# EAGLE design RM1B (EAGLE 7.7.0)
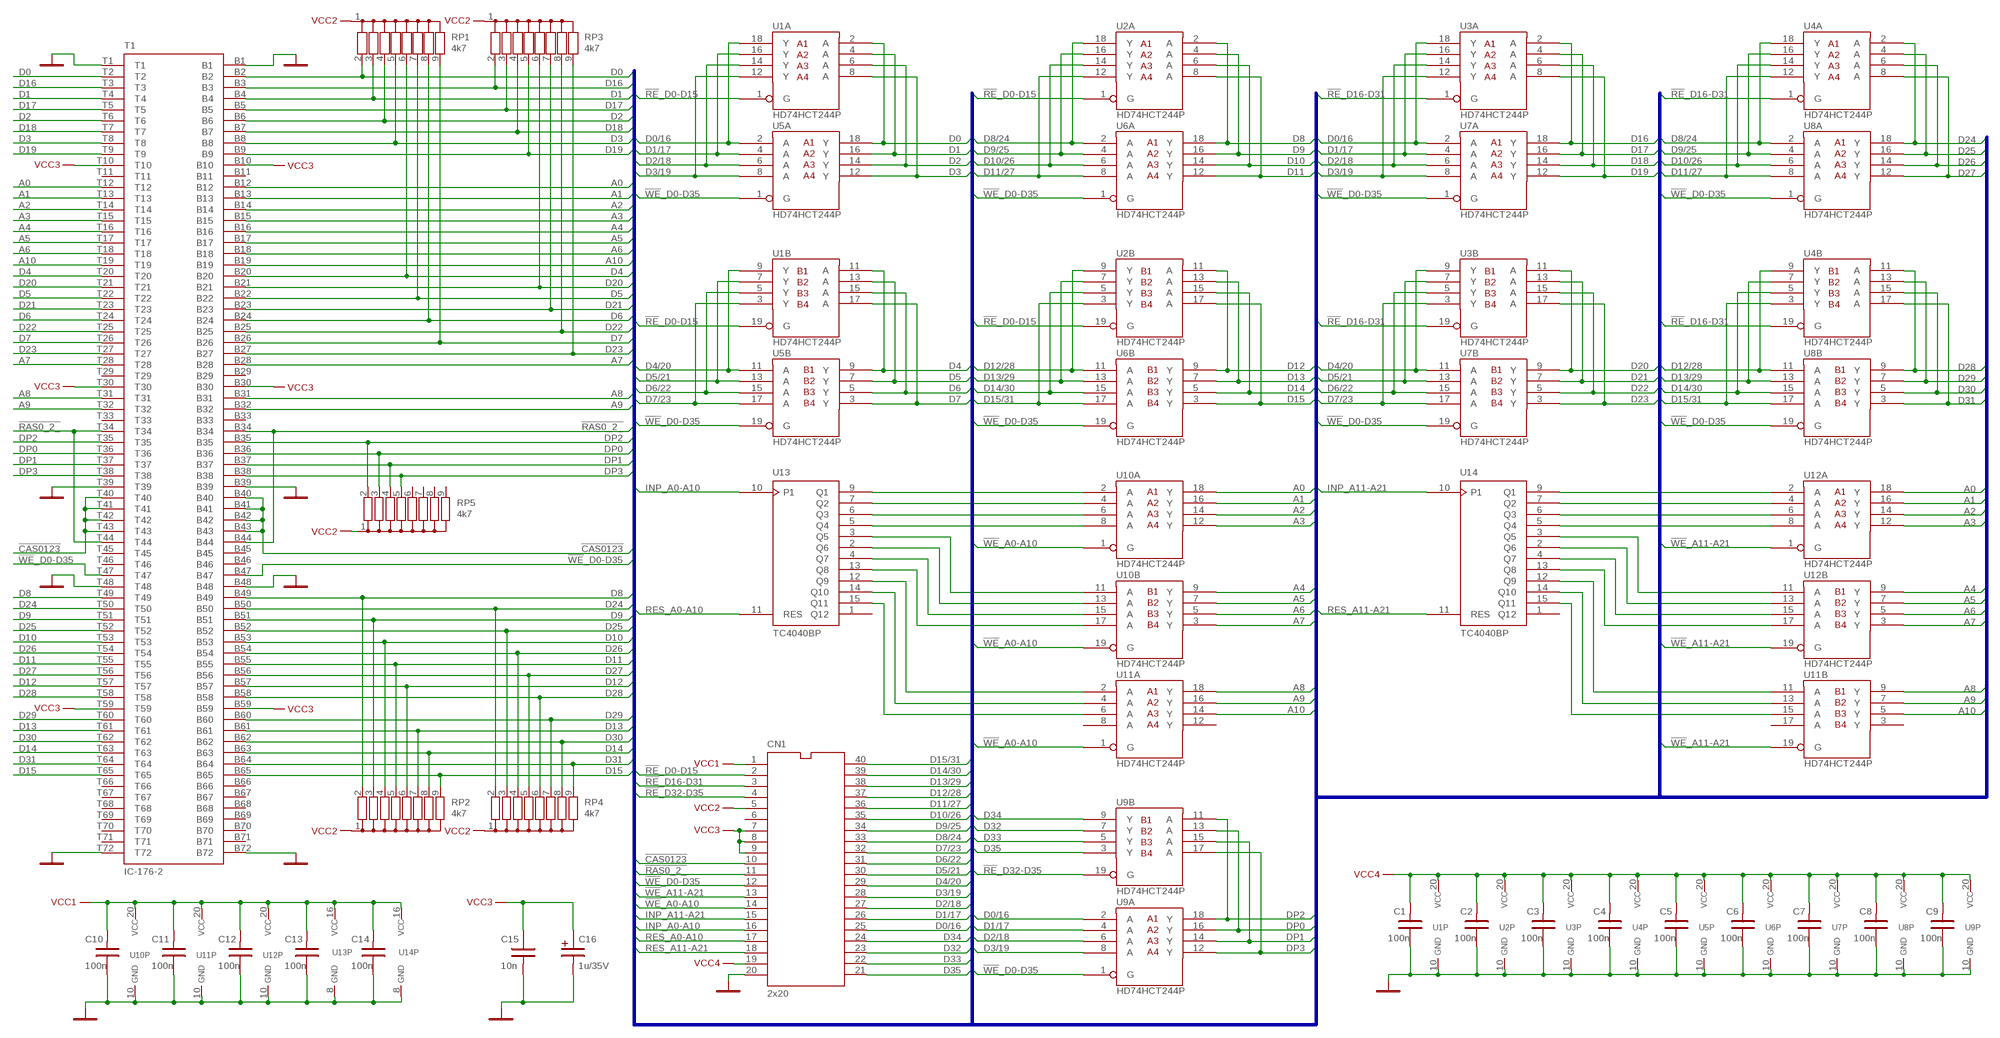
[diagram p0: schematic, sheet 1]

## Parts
C1  100n  KER-C  [KER-C]
C2  100n  KER-C  [KER-C]
C3  100n  KER-C  [KER-C]
C4  100n  KER-C  [KER-C]
C5  100n  KER-C  [KER-C]
C6  100n  KER-C  [KER-C]
C7  100n  KER-C  [KER-C]
C8  100n  KER-C  [KER-C]
C9  100n  KER-C  [KER-C]
C10  100n  KER-C  [KER-C]
C11  100n  KER-C  [KER-C]
C12  100n  KER-C  [KER-C]
C13  100n  KER-C  [KER-C]
C14  100n  KER-C  [KER-C]
C15  10n  KER-C  [KER-C]
C16  1u/35V  E-TANT-5  [E-TANT-5]
CN1  2x20  DIL40  [DIL40]
RP1  4k7  R-NET8A  [R-NET8A]
RP2  4k7  R-NET8A  [R-NET8A]
RP3  4k7  R-NET8A  [R-NET8A]
RP4  4k7  R-NET8A  [R-NET8A]
RP5  4k7  R-NET8A  [R-NET8A]
T1  IC-176-2  [IC-176-2]
U1  HD74HCT244P  74244  [DIL20]
U2  HD74HCT244P  74244  [DIL20]
U3  HD74HCT244P  74244  [DIL20]
U4  HD74HCT244P  74244  [DIL20]
U5  HD74HCT244P  74244  [DIL20]
U6  HD74HCT244P  74244  [DIL20]
U7  HD74HCT244P  74244  [DIL20]
U8  HD74HCT244P  74244  [DIL20]
U9  HD74HCT244P  74244  [DIL20]
U10  HD74HCT244P  74244  [DIL20]
U11  HD74HCT244P  74244  [DIL20]
U12  HD74HCT244P  74244  [DIL20]
U13  TC4040BP  4040  [DIL16]
U14  TC4040BP  4040  [DIL16]

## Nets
!CAS0123: CN1.10 T1.B40 T1.B41 T1.B42 T1.B43 T1.T40 T1.T41 T1.T42 T1.T43
!RAS0_2_: CN1.11 T1.B34 T1.B44 T1.T34 T1.T44
!RE!_D0-D15: CN1.2 U1.1(A:G) U1.19(B:G) U2.1(A:G) U2.19(B:G)
!RE!_D16-D31: CN1.3 U3.1(A:G) U3.19(B:G) U4.1(A:G) U4.19(B:G)
!RE!_D32-D35: CN1.4 U9.19(B:G)
!WE!_A0-A10: CN1.14 U10.1(A:G) U10.19(B:G) U11.1(A:G)
!WE!_A11-A21: CN1.13 U11.19(B:G) U12.1(A:G) U12.19(B:G)
!WE!_D0-D35: CN1.12 T1.B47 T1.T47 U5.1(A:G) U5.19(B:G) U6.1(A:G) U6.19(B:G) U7.1(A:G) U7.19(B:G) U8.1(A:G) U8.19(B:G) U9.1(A:G)
A0: T1.B12 T1.T12 U10.18(A1:Y) U12.18(A1:Y)
A1: T1.B13 T1.T13 U10.16(A2:Y) U12.16(A2:Y)
A2: T1.B14 T1.T14 U10.14(A3:Y) U12.14(A3:Y)
A3: T1.B15 T1.T15 U10.12(A4:Y) U12.12(A4:Y)
A4: T1.B16 T1.T16 U10.9(B1:Y) U12.9(B1:Y)
A5: T1.B17 T1.T17 U10.7(B2:Y) U12.7(B2:Y)
A6: T1.B18 T1.T18 U10.5(B3:Y) U12.5(B3:Y)
A7: T1.B28 T1.T28 U10.3(B4:Y) U12.3(B4:Y)
A8: T1.B31 T1.T31 U11.9(B1:Y) U11.18(A1:Y)
A9: T1.B32 T1.T32 U11.7(B2:Y) U11.16(A2:Y)
A10: T1.B19 T1.T19 U11.5(B3:Y) U11.14(A3:Y)
D0: RP1.2 T1.B2 T1.T2 U1.2(A1:A) U5.18(A1:Y)
D0/16: CN1.25 U1.18(A1:Y) U3.18(A1:Y) U5.2(A1:A) U7.2(A1:A) U9.2(A1:A)
D1: RP1.3 T1.B4 T1.T4 U1.4(A2:A) U5.16(A2:Y)
D1/17: CN1.26 U1.16(A2:Y) U3.16(A2:Y) U5.4(A2:A) U7.4(A2:A) U9.4(A2:A)
D2: RP1.4 T1.B6 T1.T6 U1.6(A3:A) U5.14(A3:Y)
D2/18: CN1.27 U1.14(A3:Y) U3.14(A3:Y) U5.6(A3:A) U7.6(A3:A) U9.6(A3:A)
D3: RP1.5 T1.B8 T1.T8 U1.8(A4:A) U5.12(A4:Y)
D3/19: CN1.28 U1.12(A4:Y) U3.12(A4:Y) U5.8(A4:A) U7.8(A4:A) U9.8(A4:A)
D4: RP1.6 T1.B20 T1.T20 U1.11(B1:A) U5.9(B1:Y)
D4/20: CN1.29 U1.9(B1:Y) U3.9(B1:Y) U5.11(B1:A) U7.11(B1:A)
D5: RP1.7 T1.B22 T1.T22 U1.13(B2:A) U5.7(B2:Y)
D5/21: CN1.30 U1.7(B2:Y) U3.7(B2:Y) U5.13(B2:A) U7.13(B2:A)
D6: RP1.8 T1.B24 T1.T24 U1.15(B3:A) U5.5(B3:Y)
D6/22: CN1.31 U1.5(B3:Y) U3.5(B3:Y) U5.15(B3:A) U7.15(B3:A)
D7: RP1.9 T1.B26 T1.T26 U1.17(B4:A) U5.3(B4:Y)
D7/23: CN1.32 U1.3(B4:Y) U3.3(B4:Y) U5.17(B4:A) U7.17(B4:A)
D8: RP2.2 T1.B49 T1.T49 U2.2(A1:A) U6.18(A1:Y)
D8/24: CN1.33 U2.18(A1:Y) U4.18(A1:Y) U6.2(A1:A) U8.2(A1:A)
D9: RP2.3 T1.B51 T1.T51 U2.4(A2:A) U6.16(A2:Y)
D9/25: CN1.34 U2.16(A2:Y) U4.16(A2:Y) U6.4(A2:A) U8.4(A2:A)
D10: RP2.4 T1.B53 T1.T53 U2.6(A3:A) U6.14(A3:Y)
D10/26: CN1.35 U2.14(A3:Y) U4.14(A3:Y) U6.6(A3:A) U8.6(A3:A)
D11: RP2.5 T1.B55 T1.T55 U2.8(A4:A) U6.12(A4:Y)
D11/27: CN1.36 U2.12(A4:Y) U4.12(A4:Y) U6.8(A4:A) U8.8(A4:A)
D12: RP2.6 T1.B57 T1.T57 U2.11(B1:A) U6.9(B1:Y)
D12/28: CN1.37 U2.9(B1:Y) U4.9(B1:Y) U6.11(B1:A) U8.11(B1:A)
D13: RP2.7 T1.B61 T1.T61 U2.13(B2:A) U6.7(B2:Y)
D13/29: CN1.38 U2.7(B2:Y) U4.7(B2:Y) U6.13(B2:A) U8.13(B2:A)
D14: RP2.8 T1.B63 T1.T63 U2.15(B3:A) U6.5(B3:Y)
D14/30: CN1.39 U2.5(B3:Y) U4.5(B3:Y) U6.15(B3:A) U8.15(B3:A)
D15: RP2.9 T1.B65 T1.T65 U2.17(B4:A) U6.3(B4:Y)
D15/31: CN1.40 U2.3(B4:Y) U4.3(B4:Y) U6.17(B4:A) U8.17(B4:A)
D16: RP3.2 T1.B3 T1.T3 U3.2(A1:A) U7.18(A1:Y)
D17: RP3.3 T1.B5 T1.T5 U3.4(A2:A) U7.16(A2:Y)
D18: RP3.4 T1.B7 T1.T7 U3.6(A3:A) U7.14(A3:Y)
D19: RP3.5 T1.B9 T1.T9 U3.8(A4:A) U7.12(A4:Y)
D20: RP3.6 T1.B21 T1.T21 U3.11(B1:A) U7.9(B1:Y)
D21: RP3.7 T1.B23 T1.T23 U3.13(B2:A) U7.7(B2:Y)
D22: RP3.8 T1.B25 T1.T25 U3.15(B3:A) U7.5(B3:Y)
D23: RP3.9 T1.B27 T1.T27 U3.17(B4:A) U7.3(B4:Y)
D24: RP4.2 T1.B50 T1.T50 U4.2(A1:A) U8.18(A1:Y)
D25: RP4.3 T1.B52 T1.T52 U4.4(A2:A) U8.16(A2:Y)
D26: RP4.4 T1.B54 T1.T54 U4.6(A3:A) U8.14(A3:Y)
D27: RP4.5 T1.B56 T1.T56 U4.8(A4:A) U8.12(A4:Y)
D28: RP4.6 T1.B58 T1.T58 U4.11(B1:A) U8.9(B1:Y)
D29: RP4.7 T1.B60 T1.T60 U4.13(B2:A) U8.7(B2:Y)
D30: RP4.8 T1.B62 T1.T62 U4.15(B3:A) U8.5(B3:Y)
D31: RP4.9 T1.B64 T1.T64 U4.17(B4:A) U8.3(B4:Y)
D32: CN1.23 U9.7(B2:Y)
D33: CN1.22 U9.5(B3:Y)
D34: CN1.24 U9.9(B1:Y)
D35: CN1.21 U9.3(B4:Y)
DP0: RP5.3 T1.B36 T1.T36 U9.13(B2:A) U9.16(A2:Y)
DP1: RP5.4 T1.B37 T1.T37 U9.14(A3:Y) U9.15(B3:A)
DP2: RP5.2 T1.B35 T1.T35 U9.11(B1:A) U9.18(A1:Y)
DP3: RP5.5 T1.B38 T1.T38 U9.12(A4:Y) U9.17(B4:A)
GND: C1.1 C2.1 C3.1 C4.1 C5.1 C6.1 C7.1 C8.1 C9.1 C10.1 C11.1 C12.1 C13.1 C14.1 C15.2 C16.K CN1.20 T1.B1 T1.B39 T1.B48 T1.B72 T1.T1 T1.T39 T1.T48 T1.T72 U1.10(P:GND) U2.10(P:GND) U3.10(P:GND) U4.10(P:GND) U5.10(P:GND) U6.10(P:GND) U7.10(P:GND) U8.10(P:GND) U9.10(P:GND) U10.10(P:GND) U11.10(P:GND) U12.10(P:GND) U13.8(GND) U14.8(GND)
INP_A0-A10: CN1.16 U13.10(P1)
INP_A11-A21: CN1.15 U14.10(P1)
N$1: U10.2(A1:A) U13.9(Q1)
N$2: U10.4(A2:A) U13.7(Q2)
N$3: U10.6(A3:A) U13.6(Q3)
N$4: U10.8(A4:A) U13.5(Q4)
N$5: U10.11(B1:A) U13.3(Q5)
N$6: U10.13(B2:A) U13.2(Q6)
N$7: U10.15(B3:A) U13.4(Q7)
N$8: U10.17(B4:A) U13.13(Q8)
N$9: U11.2(A1:A) U13.12(Q9)
N$10: U11.4(A2:A) U13.14(Q10)
N$11: U11.6(A3:A) U13.15(Q11)
N$12: U12.2(A1:A) U14.9(Q1)
N$13: U12.4(A2:A) U14.7(Q2)
N$14: U12.6(A3:A) U14.6(Q3)
N$15: U12.8(A4:A) U14.5(Q4)
N$16: U12.11(B1:A) U14.3(Q5)
N$17: U12.13(B2:A) U14.2(Q6)
N$18: U12.15(B3:A) U14.4(Q7)
N$19: U12.17(B4:A) U14.13(Q8)
N$20: U11.11(B1:A) U14.12(Q9)
N$21: U11.13(B2:A) U14.14(Q10)
N$22: U11.15(B3:A) U14.15(Q11)
RES_A0-A10: CN1.17 U13.11(RES)
RES_A11-A21: CN1.18 U14.11(RES)
VCC1: C10.2 C11.2 C12.2 C13.2 C14.2 CN1.1 U10.20(P:VCC) U11.20(P:VCC) U12.20(P:VCC) U13.16(VCC) U14.16(VCC)
VCC2: CN1.5 RP1.1 RP2.1 RP3.1 RP4.1 RP5.1
VCC3: C15.1 C16.A CN1.7 CN1.8 CN1.9 T1.B10 T1.B30 T1.B59 T1.T10 T1.T30 T1.T59
VCC4: C1.2 C2.2 C3.2 C4.2 C5.2 C6.2 C7.2 C8.2 C9.2 CN1.19 U1.20(P:VCC) U2.20(P:VCC) U3.20(P:VCC) U4.20(P:VCC) U5.20(P:VCC) U6.20(P:VCC) U7.20(P:VCC) U8.20(P:VCC) U9.20(P:VCC)
Unconnected: CN1.6 RP5.6 RP5.7 RP5.8 RP5.9 T1.B11 T1.B29 T1.B33 T1.B45 T1.B46 T1.B66 T1.B67 T1.B68 T1.B69 T1.B70 T1.B71 T1.T11 T1.T29 T1.T33 T1.T45 T1.T46 T1.T66 T1.T67 T1.T68 T1.T69 T1.T70 T1.T71 U11.3(B4:Y) U11.8(A4:A) U11.12(A4:Y) U11.17(B4:A) U13.1(Q12) U14.1(Q12)

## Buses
A[0..10],D[0..35],DP[0..3],!RE!_D0-D15,!RE!_D16-D31,!RE!_D32-D35,!CAS0123,!RAS0_2_,!WE!_D0-D35,!WE!_A11-A21,!WE!_A0-A10,INP_A11-A21,INP_A0-A10,RES_A0-A10,RES_A11-A21,D15/31,D14/30,D13/29,D12/28,D11/27,D10/26,D9/25,D8/24,D7/23,D6/22,D5/21,D4/20,D3/19,D2/18,D1/17,D0/16

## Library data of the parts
C1-C15 = PASIV:KER-C
C16 = PASIV:E-TANT-5
CN1 = SVORKY:DIL40
RP1-RP5 = PASIV:R-NET8A
T1 = CONNEC:IC-176-2
U1-U12 = 74499:74244
U13 U14 = 40XX:4040

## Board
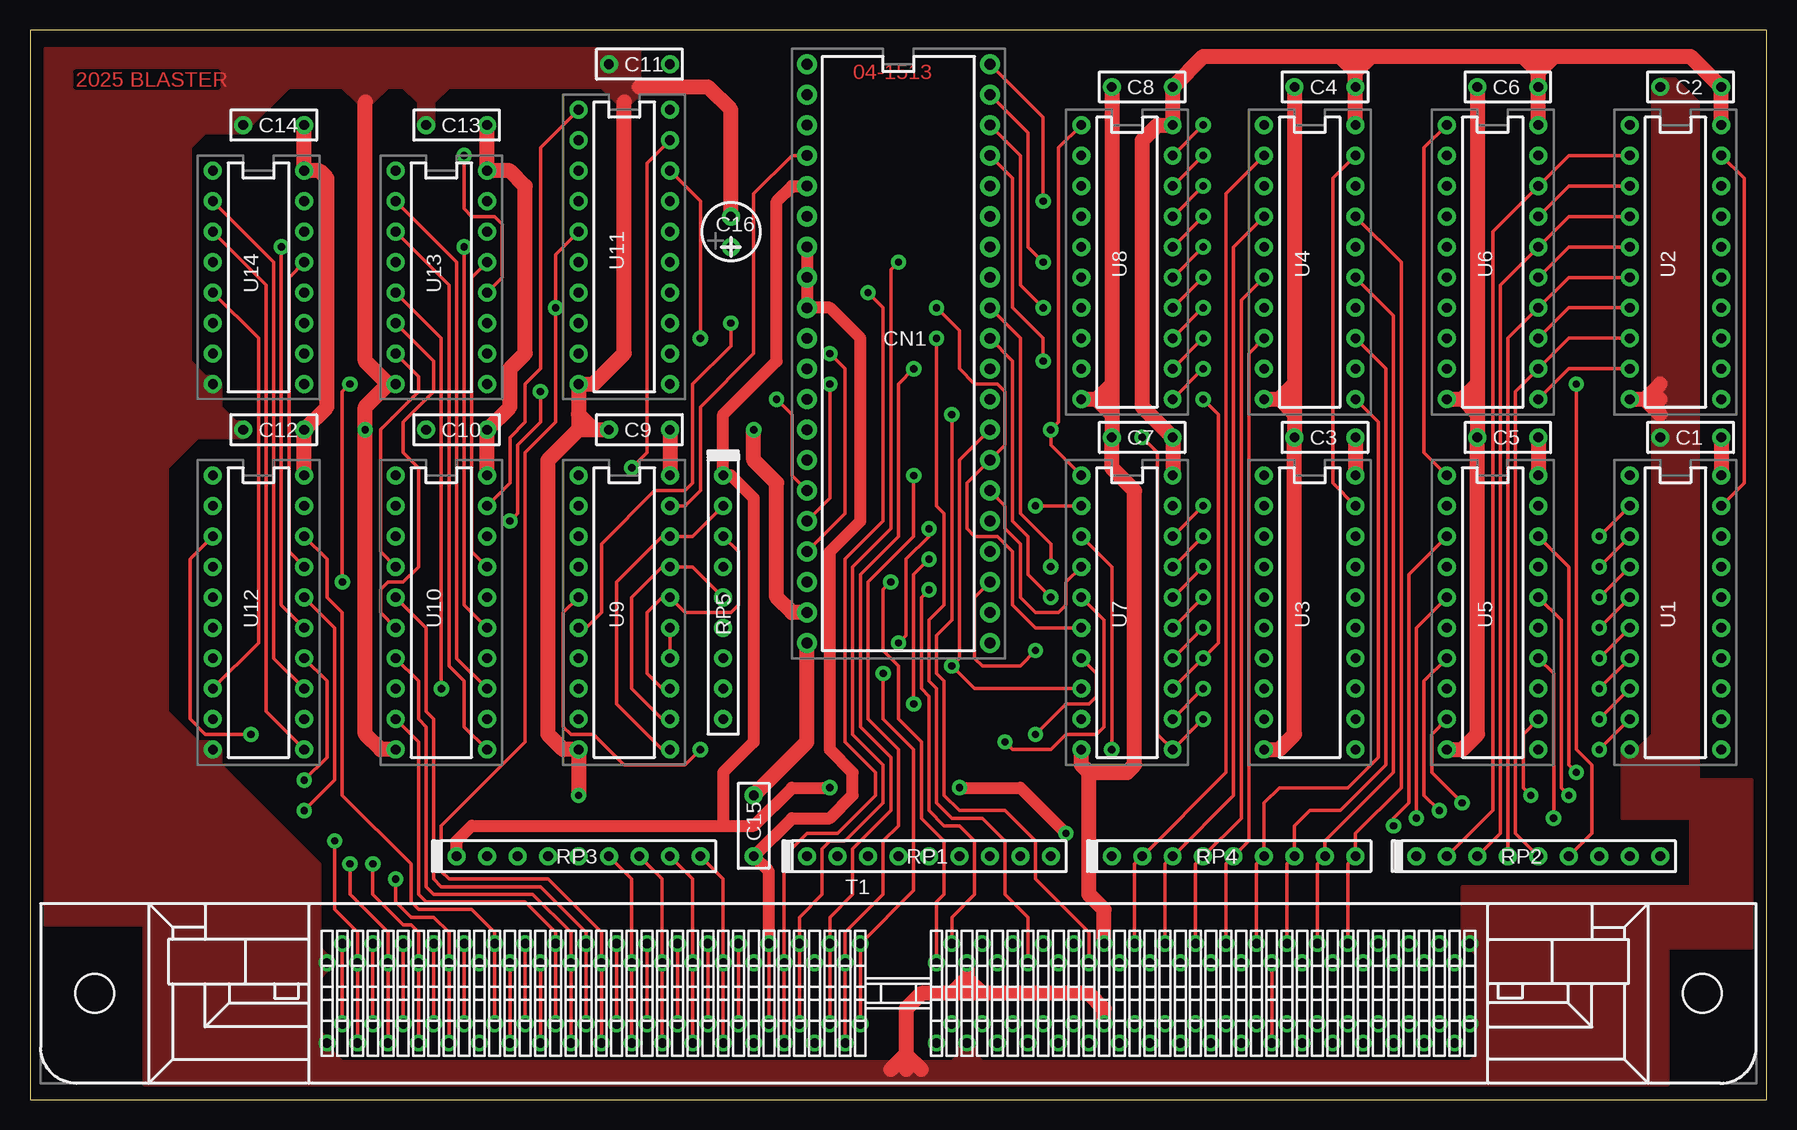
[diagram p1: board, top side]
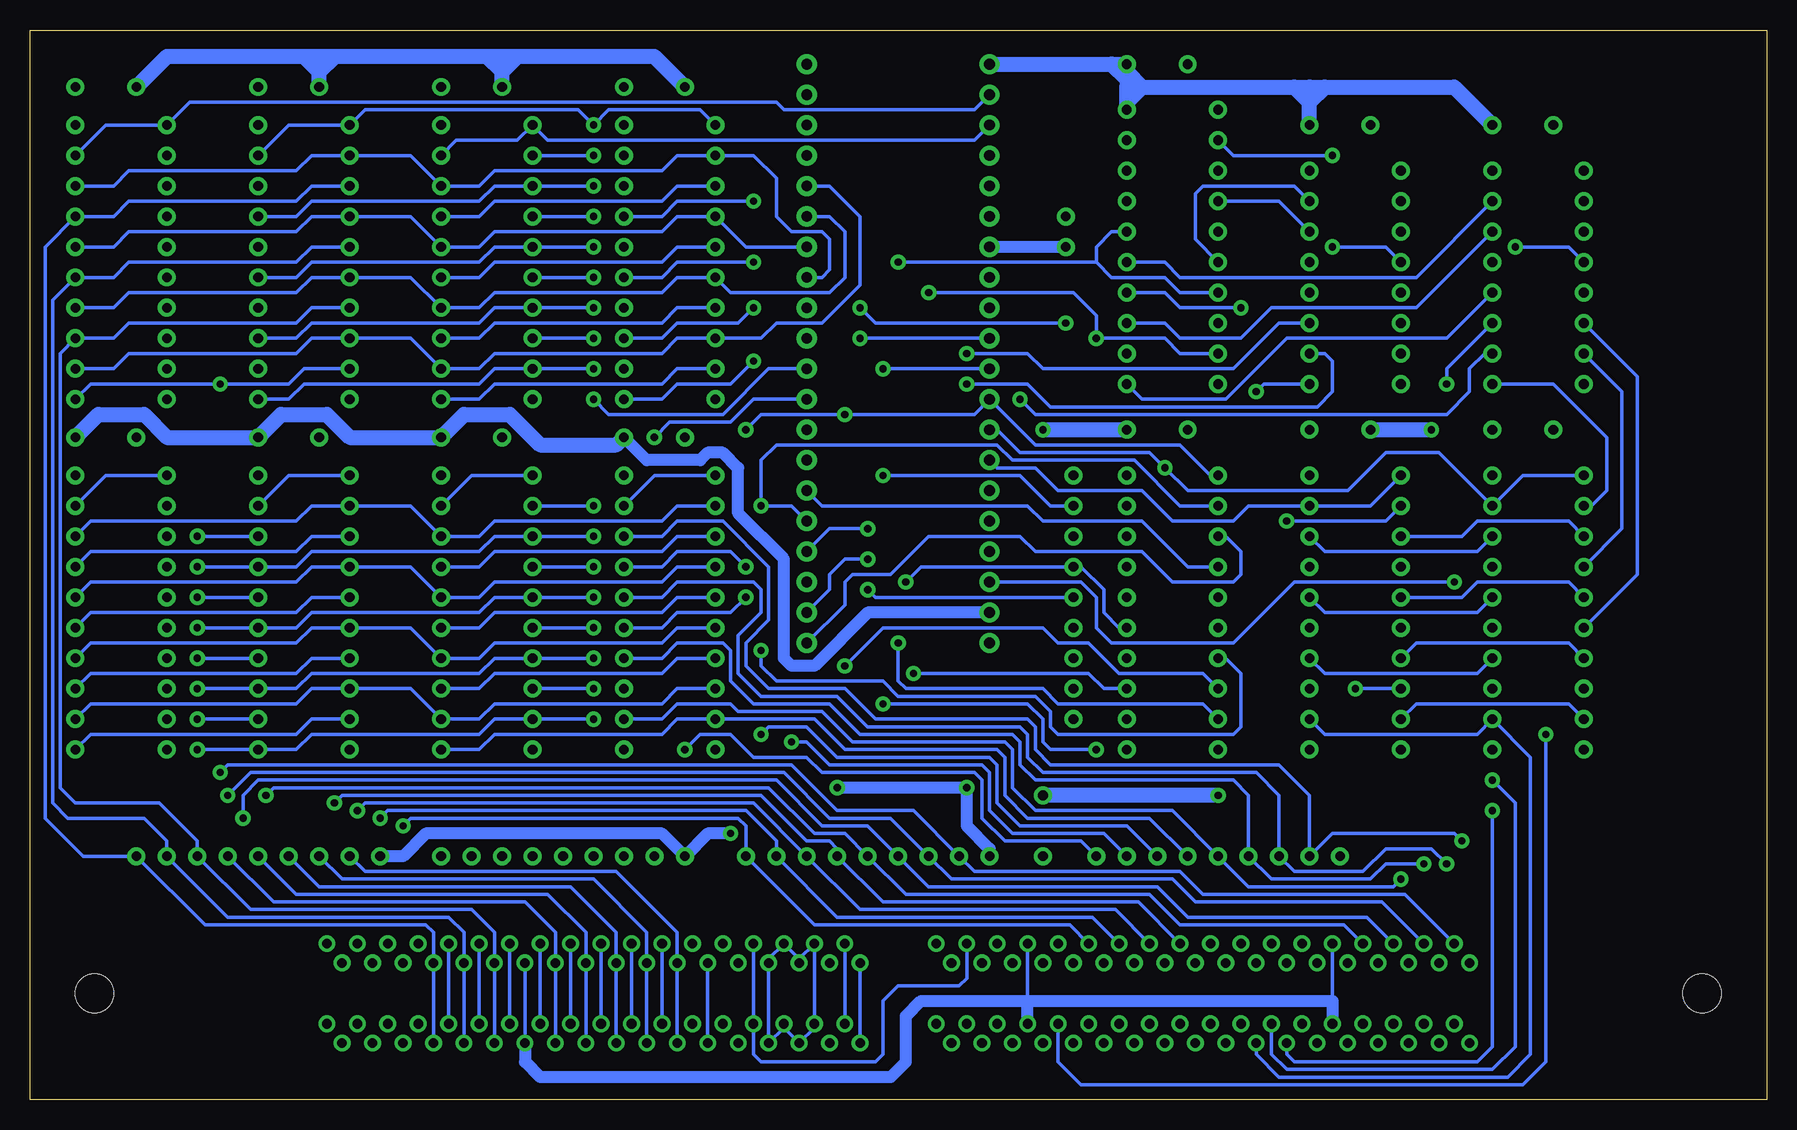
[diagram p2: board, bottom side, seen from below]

Size 144.76 x 89.2 mm. Coordinates in mm from the lower left corner, seen from the top.
Outline: 0,0 144.76,0 144.76,89.2 0,89.2 0,0
Copper layers (1*16): Top 0.035mm / dielectric 1.5mm / Bottom 0.035mm
Design rules "default *": minimum track width 10mil, minimum drill 20mil, track to track 8mil, track to pad 8mil, pad to pad 8mil, via to via 8mil, smd to smd 8mil, copper to edge 40mil, drill to drill 8mil, minimum pad ring 10mil, minimum via ring 8mil, stop-mask expansion 4mil, vias tented up to drill 0mil, thermal gap 10mil

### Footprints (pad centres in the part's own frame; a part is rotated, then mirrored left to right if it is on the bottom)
KER-C = drill 0.813 pad 1.499: 1 0,0; 2 5.08,0
E-TANT-5 = drill 0.813 pad 1.499: A -1.27,0; K 1.27,0
DIL40 = drill 0.9 pad 1.676: 1 0,0; 2 2.54,0; 3 5.08,0; 4 7.62,0; 5 10.16,0; 6 12.7,0; 7 15.24,0; 8 17.78,0; 9 20.32,0; 10 22.86,0; 11 25.4,0; 12 27.94,0; 13 30.48,0; 14 33.02,0; 15 35.56,0; 16 38.1,0; 17 40.64,0; 18 43.18,0; 19 45.72,0; 20 48.26,0; 21 48.26,15.24; 22 45.72,15.24; 23 43.18,15.24; 24 40.64,15.24; 25 38.1,15.24; 26 35.56,15.24; 27 33.02,15.24; 28 30.48,15.24; 29 27.94,15.24; 30 25.4,15.24; 31 22.86,15.24; 32 20.32,15.24; 33 17.78,15.24; 34 15.24,15.24; 35 12.7,15.24; 36 10.16,15.24; 37 7.62,15.24; 38 5.08,15.24; 39 2.54,15.24; 40 0,15.24
R-NET8A = drill 0.813 pad 1.499: 1 0,0; 2 2.54,0; 3 5.08,0; 4 7.62,0; 5 10.16,0; 6 12.7,0; 7 15.24,0; 8 17.78,0; 9 20.32,0
IC-176-2 = drill 0.8 pad 1.4: B1 -47.625,2.54; B2 -46.355,4.14; B3 -45.085,2.54; B4 -43.815,4.14; B5 -42.545,2.54; B6 -41.275,4.14; B7 -40.005,2.54; B8 -38.735,4.14; B9 -37.465,2.54; B10 -36.195,4.14; B11 -34.925,2.54; B12 -33.655,4.14; B13 -32.385,2.54; B14 -31.115,4.14; B15 -29.845,2.54; B16 -28.575,4.14; B17 -27.305,2.54; B18 -26.035,4.14; B19 -24.765,2.54; B20 -23.495,4.14; B21 -22.225,2.54; B22 -20.955,4.14; B23 -19.685,2.54; B24 -18.415,4.14; B25 -17.145,2.54; B26 -15.875,4.14; B27 -14.605,2.54; B28 -13.335,4.14; B29 -12.065,2.54; B30 -10.795,4.14; B31 -9.525,2.54; B32 -8.255,4.14; B33 -6.985,2.54; B34 -5.715,4.14; B35 -4.445,2.54; B36 -3.175,4.14; B37 3.175,2.54; B38 4.445,4.14; B39 5.715,2.54; B40 6.985,4.14; B41 8.255,2.54; B42 9.525,4.14; B43 10.795,2.54; B44 12.065,4.14; B45 13.335,2.54; B46 14.605,4.14; B47 15.875,2.54; B48 17.145,4.14; B49 18.415,2.54; B50 19.685,4.14; B51 20.955,2.54; B52 22.225,4.14; B53 23.495,2.54; B54 24.765,4.14; B55 26.035,2.54; B56 27.305,4.14; B57 28.575,2.54; B58 29.845,4.14; B59 31.115,2.54; B60 32.385,4.14; B61 33.655,2.54; B62 34.925,4.14; B63 36.195,2.54; B64 37.465,4.14; B65 38.735,2.54; B66 40.005,4.14; B67 41.275,2.54; B68 42.545,4.14; B69 43.815,2.54; B70 45.085,4.14; B71 46.355,2.54; B72 47.625,4.14; T1 -47.625,-4.14; T2 -46.355,-2.54; T3 -45.085,-4.14; T4 -43.815,-2.54; T5 -42.545,-4.14; T6 -41.275,-2.54; T7 -40.005,-4.14; T8 -38.735,-2.54; T9 -37.465,-4.14; T10 -36.195,-2.54; T11 -34.925,-4.14; T12 -33.655,-2.54; T13 -32.385,-4.14; T14 -31.115,-2.54; T15 -29.845,-4.14; T16 -28.575,-2.54; T17 -27.305,-4.14; T18 -26.035,-2.54; T19 -24.765,-4.14; T20 -23.495,-2.54; T21 -22.225,-4.14; T22 -20.955,-2.54; T23 -19.685,-4.14; T24 -18.415,-2.54; T25 -17.145,-4.14; T26 -15.875,-2.54; T27 -14.605,-4.14; T28 -13.335,-2.54; T29 -12.065,-4.14; T30 -10.795,-2.54; T31 -9.525,-4.14; T32 -8.255,-2.54; T33 -6.985,-4.14; T34 -5.715,-2.54; T35 -4.445,-4.14; T36 -3.175,-2.54; T37 3.175,-4.14; T38 4.445,-2.54; T39 5.715,-4.14; T40 6.985,-2.54; T41 8.255,-4.14; T42 9.525,-2.54; T43 10.795,-4.14; T44 12.065,-2.54; T45 13.335,-4.14; T46 14.605,-2.54; T47 15.875,-4.14; T48 17.145,-2.54; T49 18.415,-4.14; T50 19.685,-2.54; T51 20.955,-4.14; T52 22.225,-2.54; T53 23.495,-4.14; T54 24.765,-2.54; T55 26.035,-4.14; T56 27.305,-2.54; T57 28.575,-4.14; T58 29.845,-2.54; T59 31.115,-4.14; T60 32.385,-2.54; T61 33.655,-4.14; T62 34.925,-2.54; T63 36.195,-4.14; T64 37.465,-2.54; T65 38.735,-4.14; T66 40.005,-2.54; T67 41.275,-4.14; T68 42.545,-2.54; T69 43.815,-4.14; T70 45.085,-2.54; T71 46.355,-4.14; T72 47.625,-2.54 | hole 3.2: -67,0; 67,0
DIL20 = drill 0.813 pad 1.499: 1 0,0; 2 2.54,0; 3 5.08,0; 4 7.62,0; 5 10.16,0; 6 12.7,0; 7 15.24,0; 8 17.78,0; 9 20.32,0; 10 22.86,0; 11 22.86,7.62; 12 20.32,7.62; 13 17.78,7.62; 14 15.24,7.62; 15 12.7,7.62; 16 10.16,7.62; 17 7.62,7.62; 18 5.08,7.62; 19 2.54,7.62; 20 0,7.62
DIL16 = drill 0.813 pad 1.499: 1 0,0; 2 2.54,0; 3 5.08,0; 4 7.62,0; 5 10.16,0; 6 12.7,0; 7 15.24,0; 8 17.78,0; 9 17.78,7.62; 10 15.24,7.62; 11 12.7,7.62; 12 10.16,7.62; 13 7.62,7.62; 14 5.08,7.62; 15 2.54,7.62; 16 0,7.62

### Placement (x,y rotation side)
C1  135.89,55.24 0 top
C2  135.89,84.45 0 top
C3  105.41,55.24 0 top
C4  105.41,84.45 0 top
C5  120.65,55.24 0 top
C6  120.65,84.45 0 top
C7  90.17,55.24 0 top
C8  90.17,84.45 0 top
C9  48.26,55.88 0 top
C10  33.02,55.88 0 top
C11  48.26,86.36 0 top
C12  17.78,55.88 0 top
C13  33.02,81.28 0 top
C14  17.78,81.28 0 top
C15  60.33,20.32 90 top
C16  58.42,72.39 90 top
CN1  64.77,86.36 270 top
RP1  64.77,20.32 0 top
RP2  115.57,20.32 0 top
RP3  35.56,20.32 0 top
RP4  90.17,20.32 0 top
RP5  57.78,52.07 270 top
T1  72.39,8.89 0 top
U1  133.35,52.07 270 top
U2  133.35,81.28 270 top
U3  102.87,52.07 270 top
U4  102.87,81.28 270 top
U5  118.11,52.07 270 top
U6  118.11,81.28 270 top
U7  87.63,52.07 270 top
U8  87.63,81.28 270 top
U9  45.72,52.07 270 top
U10  30.48,52.07 270 top
U11  45.72,82.55 270 top
U12  15.24,52.07 270 top
U13  30.48,77.47 270 top
U14  15.24,77.47 270 top

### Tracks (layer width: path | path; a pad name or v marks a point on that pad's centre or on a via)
!CAS0123  (via drill 0.6 pad 1.27)
  Top 0.305: T1.B43 83.19,15.24 81.28,17.14 81.28,21.59 79.38,23.5 76.83,23.5 75.56,24.77 75.56,34.29 74.93,34.92 74.93,40.01 76.2,41.27 76.2,48.9 75.56,49.53 v75.56,63.5
  Bottom 0.305: T1.T42 81.92,6.02 | 81.92,6.02 T1.T43 | 81.92,6.02 T1.T41 79.38,6.02 T1.T40 T1.B40 80.64,11.76 | 80.64,11.76 T1.B42 83.19,11.76 T1.B43 83.19,4.76 | T1.B41 80.64,11.76 | v75.56,63.5 CN1.10
!RAS0_2_  (via drill 0.6 pad 1.27)
  Top 0.305: T1.T34 T1.B34 66.67,15.24 68.58,17.14 68.58,20.95 71.75,24.13 71.75,28.57 69.22,31.11 69.22,43.81 72.39,46.99 72.39,59.69 v73.66,60.96
  Bottom 0.305: T1.B44 T1.T44 84.45,3.81 83.82,3.17 74.3,3.17 73.66,3.81 73.66,8.26 72.39,9.53 67.31,9.53 66.67,10.16 T1.B34 | v73.66,60.96 CN1.11
!RE!_D0-D15
  Top 0.305: U2.19 142.88,76.83 142.88,51.44 U1.19
  Bottom 0.305: U1.19 138.43,52.07 U1.1 | U2.19 138.43,81.28 U2.1 131.44,83.19 82.55,83.19 81.92,82.55 66.04,82.55 CN1.2
!RE!_D16-D31
  Top 0.305: U4.19 108.58,76.83 108.58,51.44 U3.19
  Bottom 0.305: U3.19 107.95,52.07 U3.1 | U4.19 109.22,80.01 104.14,80.01 U4.1 101.6,80.01 66.04,80.01 CN1.3
!RE!_D32-D35
  Top 0.305: CN1.4 63.5,78.74 60.33,75.56 60.33,62.23 55.88,57.78 55.88,50.8 54.61,49.53 U9.19
!WE!_A0-A10
  Top 0.305: U11.1 42.55,79.38 42.55,60.96 41.27,59.69 41.27,56.52 40.01,55.24 40.01,51.44 U10.19
  Bottom 0.305: U10.1 33.02,49.53 U10.19 43.18,49.53 44.45,48.26 49.53,48.26 52.07,50.8 59.05,50.8 60.96,52.7 64.14,52.7 CN1.14
!WE!_A11-A21  (via drill 0.6 pad 1.27)
  Top 0.305: U11.19 51.44,78.11 51.44,53.98 v50.16,52.7
  Bottom 0.305: CN1.13 64.14,55.88 62.23,53.98 51.44,53.98 v50.16,52.7 48.26,50.8 34.92,50.8 31.75,53.98 27.3,53.98 U12.19 20.32,52.07 U12.1
!WE!_D0-D35  (via drill 0.6 pad 1.27)
  Top 0.305: U6.1 116.2,79.38 116.2,53.98 U5.1 | U8.19 v97.79,81.28 | U8.1 85.72,79.38 85.72,56.52 v85.09,55.88 85.09,54.61 U7.1 | T1.B47 88.27,13.97 83.82,18.41 83.82,21.59 81.28,24.13 77.47,24.13 76.2,25.4 76.2,34.92 75.56,35.56 75.56,38.73 76.83,40.01 v76.83,57.15
  Bottom 0.305: T1.T47 T1.B47 | U6.19 123.19,81.28 U6.1 116.84,82.55 99.06,82.55 v97.79,81.28 96.52,82.55 88.9,82.55 U8.1 | U5.19 123.19,52.07 U5.1 | U7.19 92.71,52.07 U7.1 | v85.09,55.88 83.82,57.15 v76.83,57.15 66.04,57.15 CN1.12 60.96,54.61 48.9,54.61 46.35,52.07 U9.1
A0
  Top 0.305: T1.T12 T1.B12 38.73,13.97 36.83,15.88 32.38,15.88 31.75,16.51 31.75,19.68 26.04,25.4 26.04,40.64 24.77,41.91 24.77,45.09 U12.18
  Bottom 0.305: U10.18 36.83,45.72 24.13,45.72 U12.18
A1  (via drill 0.6 pad 1.27)
  Top 0.305: T1.T13 T1.B13 | U12.16 25.4,39.37 25.4,26.67 v22.86,24.13
  Bottom 0.305: v22.86,24.13 22.86,4.45 24.13,3.17 39.37,3.17 40.01,3.81 T1.T13 | U10.16 36.83,40.64 24.13,40.64 U12.16
A2  (via drill 0.6 pad 1.27)
  Top 0.305: T1.T14 T1.B14 | U12.14 24.77,34.92 24.77,28.57 v22.86,26.67
  Bottom 0.305: v22.86,26.67 20.95,24.77 20.95,4.45 22.86,2.54 40.01,2.54 41.27,3.81 T1.T14 | U10.14 36.83,35.56 24.13,35.56 U12.14
A3
  Top 0.305: T1.T15 T1.B15
  Bottom 0.305: T1.T15 42.55,3.81 40.64,1.91 21.59,1.91 19.68,3.81 19.68,28.57 U12.12 24.13,30.48 36.83,30.48 U10.12
A4
  Top 0.305: T1.T16 T1.B16 43.81,13.97 41.27,16.51 33.02,16.51 32.38,17.14 32.38,29.84 U10.9
  Bottom 0.305: U10.9 29.21,33.02 16.51,33.02 U12.9
A5
  Top 0.305: T1.T17 T1.B17 45.09,13.97 41.91,17.14 33.66,17.14 33.02,17.78 33.02,31.11 32.38,31.75 32.38,34.92 U10.7
  Bottom 0.305: U10.7 29.21,38.1 16.51,38.1 U12.7
A6
  Top 0.305: T1.T18 T1.B18 46.35,13.97 42.55,17.78 34.29,17.78 33.66,18.41 33.66,31.75 33.02,32.38 33.02,39.37 U10.5
  Bottom 0.305: U10.5 25.4,41.91 24.13,43.18 16.51,43.18 U12.5
A7  (via drill 0.6 pad 1.27)
  Top 0.305: T1.T28 T1.B28 | U12.3 13.34,45.09 13.34,31.75 14.61,30.48 v18.41,30.48
  Bottom 0.305: v18.41,30.48 18.41,3.17 20.32,1.27 57.15,1.27 59.05,3.17 T1.T28 | U10.3 25.4,46.99 24.13,48.26 16.51,48.26 U12.3
A8  (via drill 0.6 pad 1.27)
  Top 0.305: T1.T31 T1.B31 62.87,20.32 64.77,22.23 67.31,22.23 70.48,25.4 70.48,27.3 67.94,29.84 67.94,45.09 71.12,48.26 71.12,66.04 v69.85,67.31 | U11.18 55.88,74.93 v55.88,63.5
  Bottom 0.305: U11.9 48.9,62.23 50.16,63.5 v55.88,63.5 55.88,65.41 57.78,67.31 v69.85,67.31
A9  (via drill 0.6 pad 1.27)
  Top 0.305: T1.T32 T1.B32 64.14,15.24 66.04,17.14 66.04,20.95 66.67,21.59 67.94,21.59 71.12,24.77 71.12,27.94 68.58,30.48 68.58,44.45 71.75,47.62 71.75,69.22 v72.39,69.85
  Bottom 0.305: v72.39,69.85 55.88,69.85 | 55.88,69.85 55.88,71.12 54.61,72.39 U11.16 | U11.7 48.9,67.31 50.16,68.58 54.61,68.58 55.88,69.85
A10  (via drill 0.6 pad 1.27)
  Top 0.305: T1.T19 T1.B19 47.62,13.97 43.18,18.41 34.92,18.41 34.29,19.05 34.29,22.86 41.27,29.84 41.27,53.98 43.81,56.52 v43.81,66.04 43.81,70.48 U11.5
  Bottom 0.305: U11.14 50.16,67.31 48.9,66.04 v43.81,66.04
D0  (via drill 0.6 pad 1.27)
  Top 0.305: T1.B2 T1.T2 | U1.2 v130.81,46.99 | U5.18 128.27,44.45 128.27,27.94 v128.91,27.3
  Bottom 0.305: v130.81,46.99 U5.18 | v128.91,27.3 128.27,27.94 81.28,27.94 77.47,24.13 71.12,24.13 RP1.2 66.04,19.05 48.9,19.05 46.99,17.14 30.15,17.14 T1.B2
D0/16  (via drill 0.6 pad 1.27)
  Top 0.305: U7.2 v83.82,49.53
  Bottom 0.305: CN1.25 81.28,49.53 v83.82,49.53 83.82,53.34 82.55,54.61 64.14,54.61 62.87,53.34 52.7,53.34 48.9,49.53 U9.2 | U1.18 139.7,48.26 122.56,48.26 121.28,49.53 U5.2 113.03,49.53 U3.18 107.31,46.99 106.05,48.26 92.08,48.26 90.81,49.53 U7.2
D1  (via drill 0.6 pad 1.27)
  Top 0.305: T1.T4 T1.B4 | U1.4 v130.81,41.91 | U5.16 127.64,40.01 127.64,26.04 v128.27,25.4
  Bottom 0.305: v130.81,41.91 U5.16 | v128.27,25.4 126.36,27.3 81.92,27.3 78.11,23.5 73.03,23.5 RP1.3 67.94,18.41 49.53,18.41 47.62,16.51 32.05,16.51 T1.B4
D1/17
  Top 0.305: CN1.26 81.28,49.53 81.28,47.62 82.55,46.35 82.55,41.91 83.82,40.64 85.72,40.64 86.36,41.27 86.36,43.18 U7.4
  Bottom 0.305: U1.16 139.7,43.18 122.56,43.18 121.28,44.45 U5.4 113.03,44.45 U3.16 107.31,41.91 106.05,43.18 92.08,43.18 90.81,44.45 U7.4 | CN1.26 78.74,49.53 61.59,49.53 60.33,48.26 52.07,48.26 48.26,44.45 U9.4
D2  (via drill 0.6 pad 1.27)
  Top 0.305: T1.T6 T1.B6 | U5.14 127,35.56 v127,23.5 | U1.6 v130.81,36.83
  Bottom 0.305: v130.81,36.83 U5.14 | v127,23.5 127,25.4 125.73,26.67 82.55,26.67 78.74,22.86 74.93,22.86 RP1.4 69.85,17.78 50.8,17.78 48.26,15.24 33.33,15.24 T1.B6
D2/18  (via drill 0.6 pad 1.27)
  Top 0.305: U9.6 46.35,39.37 47.62,40.64 47.62,46.35 52.07,50.8 54.61,50.8 55.24,51.44 55.24,59.69 58.42,62.87 v58.42,64.77 | U7.6 83.82,39.37 81.92,41.27 81.92,45.72 80.64,46.99 78.74,46.99 78.11,47.62 78.11,51.44 CN1.27 81.28,54.61 81.28,59.05 80.64,59.69 78.74,59.69 77.47,60.96 77.47,64.14 v75.56,66.04
  Bottom 0.305: U1.14 139.7,38.1 122.56,38.1 121.28,39.37 U5.6 113.03,39.37 U3.14 107.31,36.83 106.05,38.1 92.08,38.1 90.81,39.37 U7.6 | v75.56,66.04 74.3,64.77 v58.42,64.77
D3  (via drill 0.6 pad 1.27)
  Top 0.305: T1.T8 T1.B8 | U1.8 v130.81,31.75 | U5.12 124.46,30.48 124.46,26.04 v125.09,25.4
  Bottom 0.305: v130.81,31.75 U5.12 | v125.09,25.4 124.46,26.04 83.19,26.04 79.38,22.23 76.83,22.23 RP1.5 71.75,17.14 51.44,17.14 48.9,14.61 35.23,14.61 T1.B8
D3/19  (via drill 0.6 pad 1.27)
  Top 0.305: U7.8 78.74,34.29 v76.83,36.2 77.47,36.83 77.47,53.34 CN1.28
  Bottom 0.305: U9.8 46.99,35.56 53.98,35.56 56.52,38.1 59.05,38.1 60.33,39.37 73.66,39.37 v76.83,36.2 | U1.12 139.7,33.02 122.56,33.02 121.28,34.29 U5.8 113.03,34.29 U3.12 107.31,31.75 106.05,33.02 92.08,33.02 90.81,34.29 U7.8
D4  (via drill 0.6 pad 1.27)
  Top 0.305: T1.T20 T1.B20 | U5.9 116.84,30.48 116.84,27.3 v119.38,24.77
  Bottom 0.305: v119.38,24.77 118.75,25.4 83.82,25.4 80.01,21.59 78.11,21.59 77.47,20.95 RP1.6 73.66,16.51 52.38,16.51 T1.B20 | U1.11 139.7,30.48 122.56,30.48 121.28,31.75 U5.9
D4/20  (via drill 0.6 pad 1.27)
  Top 0.305: v130.81,29.21 U1.9 | v97.79,31.75 U7.11 93.98,30.48 93.98,53.98 v92.71,55.24
  Bottom 0.305: v130.81,29.21 U5.11 122.56,29.21 121.28,30.48 107.31,30.48 106.05,31.75 U3.9 v97.79,31.75 | v92.71,55.24 91.44,56.52 86.36,56.52 84.45,58.42 CN1.29
D5  (via drill 0.6 pad 1.27)
  Top 0.305: T1.T22 T1.B22 | U5.7 116.2,34.92 116.2,25.4 v117.47,24.13
  Bottom 0.305: v117.47,24.13 116.84,24.77 84.45,24.77 RP1.7 75.56,15.88 54.28,15.88 T1.B22 | U1.13 139.7,35.56 122.56,35.56 121.28,36.83 U5.7
D5/21  (via drill 0.6 pad 1.27)
  Top 0.305: v130.81,34.29 U1.7 | U7.13 v97.79,36.83 99.06,38.1 99.06,57.15 v97.79,58.42
  Bottom 0.305: v130.81,34.29 U5.13 122.56,34.29 121.28,35.56 107.31,35.56 106.05,36.83 U3.7 v97.79,36.83 | v97.79,58.42 96.52,57.15 87,57.15 83.19,60.96 CN1.30
D6  (via drill 0.6 pad 1.27)
  Top 0.305: T1.T24 T1.B24 | U5.5 115.57,39.37 v115.57,23.5
  Bottom 0.305: v115.57,23.5 114.94,24.13 85.09,24.13 82.55,21.59 RP1.8 77.47,15.24 56.19,15.24 T1.B24 | U1.15 139.7,40.64 122.56,40.64 121.28,41.91 U5.5
D6/22  (via drill 0.6 pad 1.27)
  Top 0.305: v130.81,39.37 U1.5 | U7.15 v97.79,41.91 | CN1.31 81.92,61.59 81.92,48.26 83.19,46.99 83.19,43.81 v85.09,41.91
  Bottom 0.305: v130.81,39.37 U5.15 122.56,39.37 121.28,40.64 107.31,40.64 106.05,41.91 U3.5 v97.79,41.91 | v85.09,41.91 86.36,40.64 90.81,40.64 92.08,39.37 U7.15
D7  (via drill 0.6 pad 1.27)
  Top 0.305: T1.T26 T1.B26 | U5.3 114.94,43.81 114.94,24.77 113.67,23.5 v113.67,22.86
  Bottom 0.305: v113.67,22.86 113.03,23.5 85.72,23.5 85.09,22.86 RP1.9 79.38,14.61 58.09,14.61 T1.B26 | U1.17 139.7,45.72 122.56,45.72 121.28,46.99 U5.3
D7/23  (via drill 0.6 pad 1.27)
  Top 0.305: v130.81,44.45 U1.3 | U7.17 v97.79,46.99 | CN1.32 82.55,63.5 82.55,48.9 85.09,46.35 v85.09,44.45
  Bottom 0.305: v130.81,44.45 U5.17 122.56,44.45 121.28,45.72 107.31,45.72 106.05,46.99 U3.3 v97.79,46.99 | v85.09,44.45 86.36,45.72 90.81,45.72 92.08,44.45 U7.17
D8
  Top 0.305: U2.2 128.27,78.74 U6.18 121.92,72.39 121.92,24.13 RP2.2
  Bottom 0.305: T1.T49 T1.B49 90.81,13.97 95.89,19.05 116.84,19.05 RP2.2
D8/24
  Bottom 0.305: U2.18 137.79,76.2 136.53,77.47 122.56,77.47 121.28,78.74 U6.2 113.03,78.74 U4.18 107.31,76.2 106.05,77.47 92.08,77.47 90.81,78.74 U8.2 84.45,78.74 82.55,76.83 82.55,73.66 81.28,72.39 78.74,72.39 78.11,71.75 78.11,69.22 78.74,68.58 CN1.33
D9
  Top 0.305: U2.4 128.27,73.66 U6.16 122.56,67.94 122.56,22.23 RP2.3
  Bottom 0.305: T1.T51 T1.B51 93.34,13.97 97.79,18.41 118.75,18.41 RP2.3
D9/25
  Bottom 0.305: U2.16 137.79,71.12 136.53,72.39 122.56,72.39 121.28,73.66 U6.4 113.03,73.66 U4.16 107.31,71.12 106.05,72.39 92.08,72.39 90.81,73.66 U8.4 85.09,71.12 CN1.34
D10
  Top 0.305: U2.6 128.27,68.58 U6.14 123.19,63.5 RP2.4
  Bottom 0.305: T1.T53 T1.B53 95.89,13.97 99.69,17.78 120.65,17.78 RP2.4
D10/26
  Bottom 0.305: U2.14 137.79,66.04 136.53,67.31 122.56,67.31 121.28,68.58 U6.6 113.03,68.58 U4.14 107.31,66.04 106.05,67.31 92.08,67.31 90.81,68.58 U8.6 86.36,67.31 78.11,67.31 76.83,68.58 76.83,72.39 78.11,73.66 CN1.35
D11
  Top 0.305: U2.8 128.27,63.5 U6.12 123.83,59.05 123.83,22.23 RP2.5
  Bottom 0.305: T1.T55 T1.B55 98.42,13.97 101.6,17.14 122.56,17.14 RP2.5
D11/27
  Bottom 0.305: U2.12 137.79,60.96 136.53,62.23 122.56,62.23 121.28,63.5 U6.8 113.03,63.5 U4.12 107.31,60.96 106.05,62.23 92.08,62.23 90.81,63.5 U8.8 83.82,63.5 82.55,64.77 78.74,64.77 75.56,67.94 75.56,73.66 78.11,76.2 CN1.36
D12  (via drill 0.6 pad 1.27)
  Top 0.305: RP2.6 130.18,22.23 130.18,27.94 128.91,29.21 v128.91,59.69
  Bottom 0.305: T1.T57 T1.B57 100.97,13.97 103.5,16.51 124.46,16.51 RP2.6 | U2.11 139.7,59.69 v128.91,59.69 123.19,59.69 121.92,60.96 U6.9
D12/28  (via drill 0.6 pad 1.27)
  Top 0.305: U6.11 128.27,60.96 U2.9 | U8.11 v97.79,60.96 | CN1.37 81.92,76.83 81.92,66.04 84.45,63.5 v84.45,61.59
  Bottom 0.305: v97.79,60.96 U4.9 106.05,60.96 107.31,59.69 121.92,59.69 123.19,58.42 U6.11 | v84.45,61.59 86.36,59.69 90.81,59.69 92.08,58.42 U8.11
D13
  Bottom 0.305: T1.T61 T1.B61 106.05,13.97 107.95,15.88 126.36,15.88 RP2.7 130.81,21.59 133.99,24.77 140.97,24.77 142.24,26.04 142.24,62.23 U2.13 137.79,63.5 136.53,64.77 122.56,64.77 121.28,66.04 U6.7
D13/29  (via drill 0.6 pad 1.27)
  Top 0.305: U6.13 128.27,66.04 U2.7 | U8.13 v97.79,66.04 | CN1.38 82.55,78.74 82.55,67.94 v84.45,66.04
  Bottom 0.305: v97.79,66.04 U4.7 106.05,66.04 107.31,64.77 121.28,64.77 122.56,63.5 U6.13 | v84.45,66.04 85.72,64.77 90.81,64.77 92.08,63.5 U8.13
D14
  Bottom 0.305: T1.T63 T1.B63 108.58,13.97 109.86,15.24 128.27,15.24 RP2.8 133.35,21.59 135.25,23.5 141.6,23.5 142.88,24.77 142.88,66.67 U2.15 137.79,68.58 136.53,69.85 122.56,69.85 121.28,71.12 U6.5
D14/30  (via drill 0.6 pad 1.27)
  Top 0.305: U6.15 128.27,71.12 U2.5 | U8.15 v97.79,71.12 | CN1.39 83.19,80.64 83.19,71.12 v84.45,69.85
  Bottom 0.305: U6.15 122.56,68.58 121.28,69.85 107.31,69.85 106.05,71.12 U4.5 v97.79,71.12 | v84.45,69.85 90.81,69.85 92.08,68.58 U8.15
D15
  Bottom 0.305: T1.T65 T1.B65 111.12,13.97 111.76,14.61 130.18,14.61 RP2.9 140.34,20.32 143.51,23.5 143.51,71.12 U2.17 137.79,73.66 136.53,74.93 122.56,74.93 121.28,76.2 U6.3
D15/31  (via drill 0.6 pad 1.27)
  Top 0.305: U6.17 128.27,76.2 U2.3 | U8.17 v97.79,76.2 | CN1.40 84.45,81.92 v84.45,74.93
  Bottom 0.305: U6.17 122.56,73.66 121.28,74.93 107.31,74.93 106.05,76.2 U4.3 v97.79,76.2 | v84.45,74.93 90.81,74.93 92.08,73.66 U8.17
D16  (via drill 0.6 pad 1.27)
  Top 0.305: T1.T3 T1.B3 27.3,13.97 25.4,15.88 v25.4,21.59 | U7.18 v97.79,49.53
  Bottom 0.305: v25.4,21.59 26.04,22.23 36.2,22.23 RP3.2 38.1,25.4 40.64,27.94 59.69,27.94 60.96,29.21 60.96,31.11 61.59,31.75 74.3,31.75 76.83,34.29 83.19,34.29 85.09,36.2 85.09,38.1 83.19,40.01 83.19,44.45 87,48.26 90.81,48.26 92.08,46.99 U7.18 | U3.2 v97.79,49.53
D17  (via drill 0.6 pad 1.27)
  Top 0.305: T1.T5 T1.B5 29.84,13.97 26.67,17.14 v26.67,19.68 | U7.16 v97.79,44.45
  Bottom 0.305: v26.67,19.68 27.94,20.95 31.75,20.95 33.66,19.05 39.37,19.05 RP3.3 40.64,25.4 42.55,27.3 60.33,27.3 61.59,28.57 61.59,30.48 62.23,31.11 74.93,31.11 77.47,33.66 83.82,33.66 85.72,35.56 85.72,38.73 83.82,40.64 83.82,42.55 84.45,43.18 90.81,43.18 92.08,41.91 U7.16 | U3.4 v97.79,44.45
D18  (via drill 0.6 pad 1.27)
  Top 0.305: T1.T7 T1.B7 32.38,13.97 31.75,14.61 31.11,14.61 28.57,17.14 v28.57,19.68 | U7.14 v97.79,39.37
  Bottom 0.305: v28.57,19.68 31.75,19.68 33.02,18.41 41.27,18.41 RP3.4 43.18,25.4 44.45,26.67 60.96,26.67 62.23,27.94 62.23,29.84 62.87,30.48 75.56,30.48 78.11,33.02 84.45,33.02 86.36,34.92 86.36,37.47 87,38.1 90.81,38.1 92.08,36.83 U7.14 | U3.6 v97.79,39.37
D19  (via drill 0.6 pad 1.27)
  Top 0.305: T1.T9 T1.B9 34.92,13.97 33.66,15.24 31.75,15.24 30.48,16.51 v30.48,18.41 | U7.12 v97.79,34.29
  Bottom 0.305: v30.48,18.41 31.11,17.78 43.18,17.78 RP3.5 49.53,24.13 60.96,24.13 62.87,26.04 62.87,29.21 63.5,29.84 76.2,29.84 78.74,32.38 85.72,32.38 86.36,33.02 90.81,33.02 92.08,31.75 U7.12 | U3.8 v97.79,34.29
D20
  Top 0.305: T1.T21 T1.B21 50.16,18.41 RP3.6
  Bottom 0.305: RP3.6 51.44,23.5 61.59,23.5 63.5,25.4 63.5,28.57 64.14,29.21 76.83,29.21 79.38,31.75 U7.9 90.81,31.75 92.08,30.48 106.05,30.48 107.31,29.21 U3.11
D21  (via drill 0.6 pad 1.27)
  Top 0.305: T1.T23 T1.B23 52.7,18.41 RP3.7 | U7.7 88.9,35.56 88.9,33.66 88.27,33.02 86.36,33.02 v83.82,30.48
  Bottom 0.305: RP3.7 53.34,22.86 62.23,22.86 64.14,24.77 64.14,27.94 64.77,28.57 77.47,28.57 80.01,31.11 83.19,31.11 v83.82,30.48 | U3.13 107.31,34.29 106.05,35.56 92.08,35.56 90.81,36.83 U7.7
D22  (via drill 0.6 pad 1.27)
  Top 0.305: T1.T25 T1.B25 55.24,18.41 RP3.8 | U7.5 89.53,40.01 89.53,31.11 88.9,30.48 86.36,30.48 85.09,29.21 81.92,29.21 v81.28,29.84
  Bottom 0.305: RP3.8 55.24,22.23 62.87,22.23 64.77,24.13 64.77,27.3 65.41,27.94 78.11,27.94 80.01,29.84 v81.28,29.84 | U3.15 107.31,39.37 106.05,40.64 92.08,40.64 90.81,41.91 U7.5
D23  (via drill 0.6 pad 1.27)
  Top 0.305: T1.T27 T1.B27 57.78,18.41 RP3.9 | U7.3 90.17,44.45 v90.17,29.21
  Bottom 0.305: RP3.9 57.15,21.59 63.5,21.59 65.41,23.5 65.41,26.67 66.04,27.3 78.74,27.3 80.01,28.57 84.45,28.57 86.36,30.48 88.9,30.48 v90.17,29.21 | U3.17 107.31,44.45 106.05,45.72 92.08,45.72 90.81,46.99 U7.3
D24  (via drill 0.6 pad 1.27)
  Top 0.305: T1.B50 92.08,19.68 RP4.2 99.69,27.3 99.69,75.56 U4.2 | U8.18 v97.79,78.74
  Bottom 0.305: T1.T50 T1.B50 | v97.79,78.74 U4.2
D25  (via drill 0.6 pad 1.27)
  Top 0.305: T1.B52 94.61,19.68 RP4.3 100.33,25.4 100.33,71.12 U4.4 | U8.16 v97.79,73.66
  Bottom 0.305: T1.T52 T1.B52 | v97.79,73.66 U4.4
D26  (via drill 0.6 pad 1.27)
  Top 0.305: T1.B54 97.16,19.68 RP4.4 100.97,23.5 100.97,66.67 U4.6 | U8.14 v97.79,68.58
  Bottom 0.305: T1.T54 T1.B54 | v97.79,68.58 U4.6
D27  (via drill 0.6 pad 1.27)
  Top 0.305: T1.B56 99.69,19.68 RP4.5 101.6,21.59 101.6,62.23 U4.8 | U8.12 v97.79,63.5
  Bottom 0.305: T1.T56 T1.B56 | v97.79,63.5 U4.8
D28
  Top 0.305: T1.B58 102.23,19.68 RP4.6 102.87,24.77 104.14,26.04 109.86,26.04 112.39,28.57 112.39,56.52 U4.11
  Bottom 0.305: T1.T58 T1.B58 | U4.11 107.31,58.42 106.05,59.69 92.08,59.69 90.81,60.96 U8.9
D29
  Top 0.305: T1.B60 104.78,19.68 RP4.7 105.41,22.86 106.68,24.13 109.22,24.13 113.03,27.94 113.03,60.96 U4.13
  Bottom 0.305: T1.T60 T1.B60 | U4.13 107.31,63.5 106.05,64.77 92.08,64.77 90.81,66.04 U8.7
D30
  Top 0.305: T1.B62 107.31,19.68 RP4.8 107.95,21.59 113.67,27.3 113.67,65.41 U4.15
  Bottom 0.305: T1.T62 T1.B62 | U4.15 107.31,68.58 106.05,69.85 92.08,69.85 90.81,71.12 U8.5
D31
  Top 0.305: T1.B64 109.86,19.68 RP4.9 110.49,22.23 114.3,26.04 114.3,69.85 U4.17
  Bottom 0.305: T1.T64 T1.B64 | U4.17 107.31,73.66 106.05,74.93 92.08,74.93 90.81,76.2 U8.3
D32  (via drill 0.6 pad 1.27)
  Top 0.305: CN1.23 78.74,41.91 78.74,36.83 79.38,36.2 82.55,36.2 v83.82,37.47
  Bottom 0.305: v83.82,37.47 83.82,36.2 82.55,34.92 73.66,34.92 72.39,33.66 60.96,33.66 59.69,32.38 59.69,31.11 59.05,30.48 44.45,30.48 43.81,31.11 43.81,35.56 45.09,36.83 U9.7
D33  (via drill 0.6 pad 1.27)
  Top 0.305: U9.5 44.45,40.64 44.45,31.11 45.09,30.48 46.99,30.48 49.53,27.94 54.61,27.94 v55.88,29.21 | v74.93,45.09 73.66,43.81 v73.66,33.02
  Bottom 0.305: CN1.22 78.11,42.55 78.11,43.81 76.83,45.09 v74.93,45.09 | v73.66,33.02 61.59,33.02 60.33,31.75 60.33,29.84 59.69,29.21 v55.88,29.21
D34  (via drill 0.6 pad 1.27)
  Top 0.305: v74.93,47.62 74.93,46.99 73.03,45.09 73.03,38.73 v72.39,38.1
  Bottom 0.305: CN1.24 78.11,47.62 v74.93,47.62 | v72.39,38.1 72.39,34.92 71.75,34.29 60.33,34.29 59.05,33.02 46.99,33.02 U9.9
D35
  Bottom 0.305: CN1.21 76.83,41.27 76.83,43.18 76.2,43.81 73.03,43.81 69.85,46.99 62.23,46.99 60.96,45.72 52.07,45.72 49.53,43.18 44.45,43.18 43.81,43.81 43.81,45.72 45.09,46.99 U9.3
DP0  (via drill 0.6 pad 1.27)
  Top 0.305: T1.T36 T1.B36 73.66,17.48 73.66,29.21 71.12,31.75 v71.12,35.56 | RP5.3 59.05,45.72 59.05,41.27 58.42,40.64 54.61,40.64 U9.16 52.7,41.91 51.44,40.64 51.44,35.56 52.7,34.29 U9.13
  Bottom 0.305: v71.12,35.56 56.52,35.56 55.24,34.29 U9.13
DP1  (via drill 0.6 pad 1.27)
  Top 0.305: U9.14 U9.15 | T1.B37 75.56,16.51 76.2,17.14 76.2,21.59 74.3,23.5 74.3,29.84 72.39,31.75 72.39,36.2 71.12,37.47 71.12,42.55 v71.75,43.18
  Bottom 0.305: T1.T37 T1.B37 | v71.75,43.18 70.48,44.45 RP5.4 57.15,44.45 55.24,42.55 55.24,40.64 53.98,39.37 U9.15
DP2  (via drill 0.6 pad 1.27)
  Top 0.305: T1.T35 T1.B35 67.94,13.97 71.12,17.14 71.12,21.59 72.39,22.86 72.39,29.21 69.85,31.75 69.85,43.18 73.66,46.99 v73.66,52.07 | U9.11 52.7,29.21 48.9,33.02 48.9,43.18 52.7,46.99 U9.18 55.24,46.99 RP5.2
  Bottom 0.305: v73.66,52.07 62.23,52.07 59.69,49.53 RP5.2
DP3  (via drill 0.6 pad 1.27)
  Top 0.305: U9.12 52.7,31.75 50.16,34.29 50.16,41.91 52.7,44.45 U9.17 55.24,44.45 RP5.5 | T1.B38 76.83,15.24 78.74,17.14 78.74,21.59 77.47,22.86 76.2,22.86 74.93,24.13 74.93,33.66 74.3,34.29 74.3,41.91 v74.93,42.55
  Bottom 0.305: T1.T38 T1.B38 | v74.93,42.55 74.3,41.91 RP5.5
GND  (via drill 0.6 pad 1.27)
  Top 1.27: 29.84,59.69 27.94,61.59 27.94,83.19 | U10.10 29.21,29.21 27.94,30.48 v27.94,55.88 27.94,57.78 29.84,59.69 | 29.84,59.69 U13.8 | 45.72,55.88 43.18,53.34 43.18,30.48 44.45,29.21 U9.10 v45.72,25.4 | 45.72,55.88 46.99,55.88 | 46.99,55.88 C9.1 | 45.72,57.15 U11.10 46.99,59.69 49.53,62.23 49.53,83.19 | 45.72,57.15 45.72,55.88 | C16.K 58.42,82.55 56.52,84.45 50.8,84.45 | 45.72,57.15 46.99,55.88 | C15.2 64.77,29.84 CN1.20 | C8.1 90.17,59.69 | 90.17,59.69 90.17,58.42 | 90.17,58.42 90.17,57.15 | 90.17,57.15 C7.1 90.17,52.7 92.08,50.8 92.08,27.94 91.44,27.3 88.27,27.3 | C4.1 105.41,59.69 | 105.41,59.69 105.41,58.42 | 105.41,58.42 105.41,57.15 | 105.41,57.15 C3.1 105.41,30.48 104.14,29.21 U3.10 | C6.1 120.65,59.69 | 120.65,59.69 120.65,58.42 | 120.65,58.42 120.65,57.15 | 120.65,57.15 C5.1 120.65,30.48 119.38,29.21 U5.10 | U8.10 88.9,58.42 | 88.9,58.42 90.17,58.42 | U4.10 104.14,58.42 | 104.14,58.42 105.41,58.42 | U6.10 119.38,58.42 | 119.38,58.42 120.65,58.42 | 88.9,58.42 90.17,59.69 | 88.9,58.42 90.17,57.15 | 104.14,58.42 105.41,59.69 | 104.14,58.42 105.41,57.15 | 119.38,58.42 120.65,59.69 | 119.38,58.42 120.65,57.15 | U2.10 134.62,58.42 | 134.62,58.42 135.89,58.42 | 134.62,58.42 135.89,59.69 | 134.62,58.42 135.89,57.15 | T1.B48 89.53,15.88 88.27,17.14 88.27,27.3 | 88.27,27.3 87.63,27.94 U7.10 | T1.T48 89.53,7.62 88.27,8.89 79.38,8.89 | 79.38,8.89 78.11,8.89 | 78.11,8.89 76.83,8.89 | 76.83,8.89 74.3,8.89 73.03,7.62 73.03,3.81 | 73.03,3.81 73.03,2.54 | T1.B39 78.11,10.16 | 78.11,10.16 78.11,8.89 | 78.11,10.16 76.83,8.89 | 78.11,10.16 79.38,8.89 | 73.03,3.81 74.3,2.54 | 73.03,3.81 71.75,2.54
  Bottom 1.27: C10.1 v27.94,55.88 | v45.72,25.4 C15.2 | C8.1 92.71,87 104.14,87 | 104.14,87 105.41,87 | 105.41,87 106.68,87 | 106.68,87 119.38,87 | 119.38,87 120.65,87 | 120.65,87 121.92,87 | 121.92,87 133.35,87 C2.1 | C4.1 105.41,85.72 | 105.41,85.72 105.41,87 | C6.1 120.65,85.72 | 120.65,85.72 120.65,87 | 105.41,85.72 104.14,87 | 105.41,85.72 106.68,87 | 120.65,85.72 119.38,87 | 120.65,85.72 121.92,87
  pour Top (no thermals): 50.16,83.19 50.8,83.82 50.8,87.63 1.27,87.63 1.27,14.61 9.53,14.61 9.53,1.27 136.53,1.27 136.53,12.7 143.51,12.7 143.51,26.67 139.06,26.67 139.06,83.19 137.16,85.09 135.89,85.09 135.25,84.45 135.25,30.48 133.99,29.21 132.72,29.21 132.72,23.5 138.43,23.5 138.43,17.78 119.38,17.78 119.38,13.34 120.65,12.06 120.65,6.99 120.02,6.35 120.65,5.71 120.65,3.81 120.02,3.17 79.38,3.17 78.74,3.81 78.74,4.45 78.11,5.08 77.47,4.45 77.47,3.81 76.83,3.17 26.04,3.17 24.77,4.45 24.77,5.08 24.13,5.71 24.13,10.16 24.77,10.79 24.77,12.06 24.13,12.7 24.13,19.68 15.88,27.94 15.88,29.21 15.24,29.84 13.97,29.84 11.43,32.38 11.43,52.7 13.97,55.24 17.78,55.24 17.78,56.52 17.14,56.52 15.88,57.78 15.88,59.69 15.24,60.33 14.61,60.33 13.34,61.59 13.34,79.38 14.61,80.64 17.78,80.64 21.59,84.45 26.04,84.45 27.3,83.19 28.57,83.19 29.84,84.45 31.11,84.45 32.38,83.19 32.38,81.28 33.66,81.28 33.66,83.19 34.92,84.45 47.62,84.45 48.9,83.19
INP_A0-A10  (via drill 0.6 pad 1.27)
  Top 0.305: CN1.16 66.67,50.16 v66.67,59.69
  Bottom 0.305: v66.67,59.69 61.59,59.69 59.69,57.78 37.47,57.78 36.2,59.05 36.2,61.59 36.83,62.23 U13.10
INP_A11-A21  (via drill 0.6 pad 1.27)
  Top 0.305: CN1.15 63.5,52.07 63.5,57.15 v62.23,58.42
  Bottom 0.305: v62.23,58.42 60.96,57.15 26.67,57.15 24.77,59.05 24.77,60.96 23.5,62.23 U14.10
N$1  (via drill 0.6 pad 1.27)
  Top 0.305: v42.55,59.05 42.55,56.52 40.64,54.61 40.64,48.9 v40.01,48.26
  Bottom 0.305: U10.2 31.75,48.26 v40.01,48.26 | v42.55,59.05 41.91,59.69 U13.9
N$2
  Top 0.305: U13.7 32.38,60.33 32.38,59.05 29.21,55.88 29.21,45.72 U10.4
N$3
  Top 0.305: U10.6 29.21,40.64 29.21,42.55 29.84,43.18 31.11,43.18 32.38,44.45 32.38,52.7 31.11,53.98 31.11,56.52 33.66,59.05 33.66,61.59 U13.6
N$4  (via drill 0.6 pad 1.27)
  Top 0.305: U13.5 34.29,63.5 v34.29,34.29
  Bottom 0.305: U10.8 v34.29,34.29
N$5
  Top 0.305: U10.11 36.2,31.11 36.2,34.92 34.92,36.2 34.92,67.94 U13.3
N$6
  Top 0.305: U10.13 35.56,36.83 35.56,69.85 U13.2
N$7  (via drill 0.6 pad 1.27)
  Top 0.305: U10.15 36.2,41.27 v36.2,71.12
  Bottom 0.305: U13.4 31.75,71.12 v36.2,71.12
N$8
  Top 0.305: U10.17 36.83,45.72 36.83,68.58 U13.13
N$9  (via drill 0.6 pad 1.27)
  Top 0.305: U13.12 39.37,68.58 39.37,73.03 38.73,73.66 36.83,73.66 36.2,74.3 v36.2,78.74
  Bottom 0.305: U11.2 44.45,78.74 v36.2,78.74
N$10
  Bottom 0.305: U11.4 40.64,74.93 U13.14
N$11
  Bottom 0.305: U13.15 39.37,76.2 46.99,76.2 47.62,75.56 47.62,71.75 U11.6
N$12
  Bottom 0.305: U14.9 17.78,59.69 13.34,55.24 13.34,50.8 14.61,49.53 U12.2
N$13
  Bottom 0.305: U14.7 12.06,59.05 12.06,47.62 U12.4
N$14
  Bottom 0.305: U14.6 10.79,60.33 10.79,43.81 U12.6
N$15
  Top 0.305: U14.5 19.05,63.5 19.05,38.1 U12.8
N$16
  Top 0.305: U14.3 19.68,67.94 19.68,32.38 U12.11
N$17
  Top 0.305: U14.2 20.32,69.85 20.32,36.83 U12.13
N$18  (via drill 0.6 pad 1.27)
  Top 0.305: U12.15 20.95,41.27 v20.95,71.12
  Bottom 0.305: v20.95,71.12 16.51,71.12 U14.4
N$19
  Top 0.305: U14.13 21.59,68.58 21.59,45.72 U12.17
N$20
  Bottom 0.305: U11.11 52.07,58.42 45.09,58.42 40.01,63.5 26.67,63.5 U14.12
N$21
  Bottom 0.305: U14.14 29.21,66.04 41.27,66.04 43.81,63.5 48.9,63.5 50.16,64.77 U11.13
N$22
  Bottom 0.305: U14.15 29.21,68.58 48.9,68.58 50.16,69.85 U11.15
RES_A0-A10  (via drill 0.6 pad 1.27)
  Top 0.305: CN1.17 67.94,48.9 67.94,60.96 v66.67,62.23
  Bottom 0.305: v66.67,62.23 61.59,62.23 60.33,60.96 44.45,60.96 40.64,64.77 U13.11
RES_A11-A21  (via drill 0.6 pad 1.27)
  Top 0.305: v26.67,59.69 26.04,59.05 v26.04,43.18
  Bottom 0.305: U14.11 26.67,60.96 v26.67,59.69 | CN1.18 57.15,43.18 55.88,41.91 55.88,39.37 54.61,38.1 44.45,38.1 39.37,43.18 v26.04,43.18
VCC1
  Top 1.27: C14.2 U14.16 24.13,77.47 24.77,76.83 24.77,57.78 C12.2 U12.20 | C13.2 U13.16 40.01,77.47 41.27,76.2 41.27,62.23 40.01,60.96 40.01,57.78 C10.2 U10.20
  Bottom 1.27: CN1.1 54.61,86.36 | 54.61,86.36 C11.2 53.34,85.72 | 53.34,85.72 53.34,85.09 | 53.34,85.09 53.34,84.45 | U11.20 53.34,83.19 | 53.34,83.19 53.34,84.45 | 53.34,84.45 52.07,84.45 | 52.07,84.45 39.37,84.45 | 39.37,84.45 38.1,84.45 | 38.1,84.45 36.83,84.45 | 36.83,84.45 26.04,84.45 C14.2 | C13.2 38.1,83.19 | 38.1,83.19 38.1,84.45 | 38.1,83.19 39.37,84.45 | 38.1,83.19 36.83,84.45 | 53.34,85.72 52.07,84.45 | 52.07,84.45 53.34,83.19 | 54.61,86.36 53.34,85.09
VCC2  (via drill 0.6 pad 1.27)
  Top 1.016: RP3.1 35.56,21.59 36.83,22.86 57.78,22.86 | 57.78,22.86 60.33,22.86 63.5,26.04 v66.67,26.04 | 57.78,22.86 57.78,27.3 60.33,29.84 60.33,50.16 58.42,52.07 RP5.1 57.78,57.15 62.23,61.59 62.23,74.93 63.5,76.2 CN1.5 | v77.47,26.04 82.55,26.04 v86.36,22.23
  Bottom 1.016: RP1.1 64.77,20.95 66.67,22.86 v66.67,26.04 v77.47,26.04 | v86.36,22.23 88.27,22.23 RP4.1 92.08,22.23 111.76,22.23 113.67,20.32 RP2.1
VCC3
  Top 0.305: T1.T59 T1.B59 | T1.B30 T1.T30 | T1.B10 T1.T10
  Top 1.016: T1.B30 61.59,19.05 C15.1 63.5,23.5 66.67,23.5 68.58,25.4 68.58,27.3 66.67,29.21 66.67,45.72 69.22,48.26 69.22,63.5 66.67,66.04 CN1.9 CN1.8 CN1.7
  Bottom 0.305: 103.5,4.76 T1.B59 | 61.59,8.26 T1.B30 | 36.2,8.26 T1.B10
  Bottom 1.016: C16.A CN1.7 | T1.T59 103.5,3.17 102.23,1.91 73.03,1.91 71.75,3.17 71.75,6.99 70.48,8.26 61.59,8.26 | T1.T30 61.59,8.26 | 61.59,8.26 36.2,8.26 T1.T10
VCC4  (via drill 0.6 pad 1.27)
  Top 1.27: C9.2 U9.20 | CN1.19 63.5,40.64 62.23,41.91 62.23,51.44 60.33,53.34 v60.33,55.88 | U2.20 C2.2 138.43,87 127,87 | 127,87 125.73,87 | 125.73,87 124.46,87 | 124.46,87 111.76,87 | 111.76,87 110.49,87 | 110.49,87 109.22,87 | 109.22,87 97.79,87 C8.2 U8.20 93.98,81.28 92.71,80.01 92.71,57.78 C7.2 U7.20 | 110.49,85.72 C4.2 U4.20 | 110.49,85.72 110.49,87 | U6.20 C6.2 125.73,85.72 | 125.73,85.72 125.73,87 | 110.49,85.72 109.22,87 | 110.49,85.72 111.76,87 | 125.73,85.72 124.46,87 | 125.73,85.72 127,87 | C3.2 U3.20 | C5.2 U5.20 | C1.2 U1.20
  Bottom 1.016: CN1.19 74.93,40.64 79.38,36.2 81.28,36.2 81.92,36.83 81.92,45.09 85.72,48.9 85.72,52.7 87,53.98 88.27,53.98 88.9,53.34 93.34,53.34 C7.2
  Bottom 1.27: v60.33,55.88 C9.2 | C1.2 139.06,57.15 135.25,57.15 133.35,55.24 C5.2 123.83,57.15 120.02,57.15 118.11,55.24 C3.2 108.58,57.15 104.78,57.15 102.23,54.61 95.89,54.61 C7.2

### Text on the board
Top: 04-1513 | 2025 BLASTER
tPotisk: ADP-RM1B | 2 | 72 | 1 | 71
